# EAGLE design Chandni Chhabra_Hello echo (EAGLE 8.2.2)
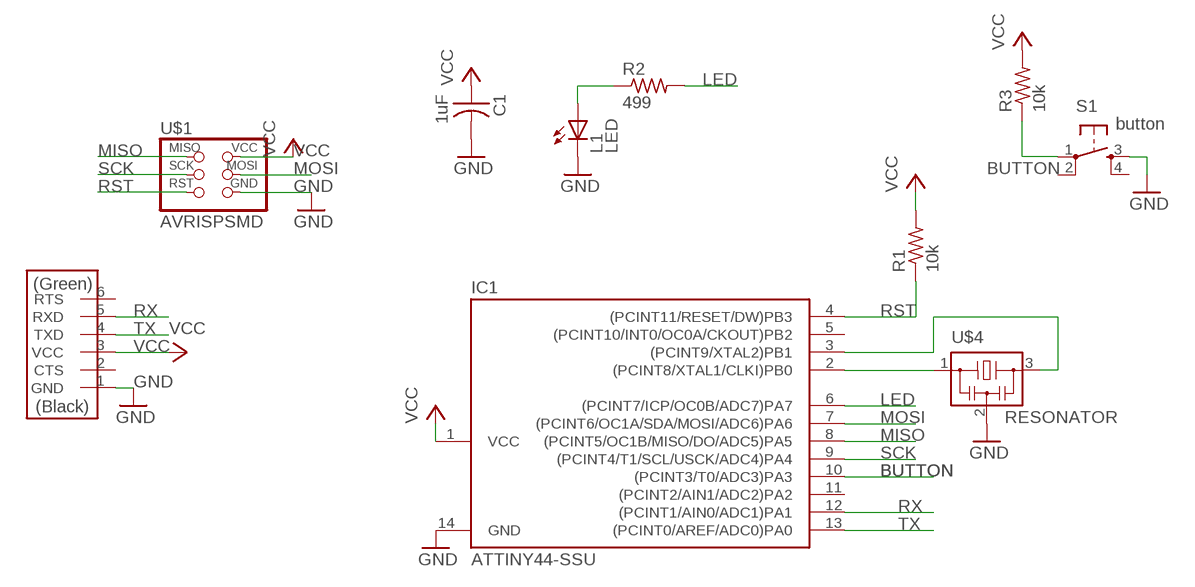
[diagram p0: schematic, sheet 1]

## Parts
C1  1uF  CAP-US1206FAB  [C1206FAB]
IC1  ATTINY44-SSU  [SOIC14]
L1  LED  [LED1206]
R1  10k  RES-US1206FAB  [R1206FAB]
R2  499  RES-US1206FAB  [R1206FAB]
R3  10k  RES-US1206FAB  [R1206FAB]
S1  button  6MM_SWITCH6MM_SWITCH  [6MM_SWITCH]
U$1  AVRISPSMD  [2X03SMD]
U$2  FTDI-SMD-HEADER  [1X06SMD]
U$4  RESONATOR  [EFOBM]

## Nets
BUTTON: IC1.10((PCINT3/T0/ADC3)PA3) R3.1 S1.1(P)
GND: C1.2 IC1.14(GND) L1.2(C) S1.3(S) U$1.6(GND) U$2.1(GND) U$4.2
LED: IC1.6((PCINT7/ICP/OC0B/ADC7)PA7) R2.2
MISO: IC1.8((PCINT5/OC1B/MISO/DO/ADC5)PA5) U$1.1(MISO)
MOSI: IC1.7((PCINT6/OC1A/SDA/MOSI/ADC6)PA6) U$1.4(MOSI)
N$1: IC1.2((PCINT8/XTAL1/CLKI)PB0) U$4.1
N$2: IC1.3((PCINT9/XTAL2)PB1) U$4.3
N$3: L1.1(A) R2.1
RST: IC1.4((PCINT11/RESET/DW)PB3) R1.1 U$1.5(RST)
RX: IC1.12((PCINT1/AIN0/ADC1)PA1) U$2.5(RXD)
SCK: IC1.9((PCINT4/T1/SCL/USCK/ADC4)PA4) U$1.3(SCK)
TX: IC1.13((PCINT0/AREF/ADC0)PA0) U$2.4(TXD)
VCC: C1.1 IC1.1(VCC) R1.2 R3.2 U$1.2(VCC) U$2.3(VCC)
Unconnected: IC1.5((PCINT10/INT0/OC0A/CKOUT)PB2) IC1.11((PCINT2/AIN1/ADC2)PA2) S1.2(P1) S1.4(S1) U$2.2(CTS) U$2.6(RTS)

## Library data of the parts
C1 = fab:CAP-US
IC1 = fab:ATTINY44
L1 = fab:LED: LED
R1-R3 = fab:RES-US: Resistor (US Symbol)
S1 = fab:6MM_SWITCH: OMRON SWITCH
U$1 = fab:AVRISP
U$2 = fab:FTDI-SMD-HEADER
U$4 = fab:RESONATOR

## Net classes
0 default: width 0.032 mm, clearance 0.4 mm

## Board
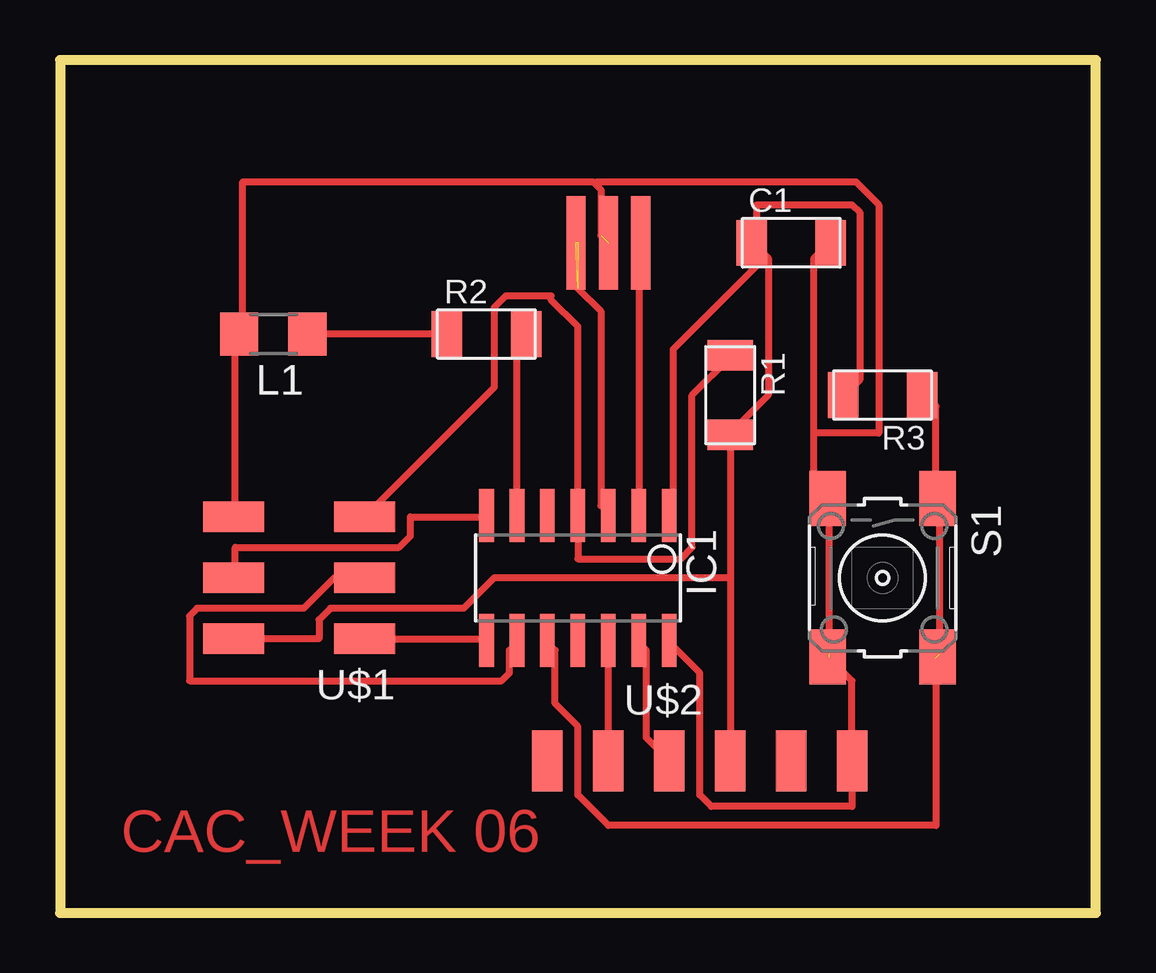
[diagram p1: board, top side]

Size 43.18 x 35.56 mm. Coordinates in mm from the lower left corner, seen from the top.
Outline: 43.18,35.56 0,35.56 0,0 43.18,0 43.18,35.56
Copper layers (1*16): Top 0.035mm / dielectric 1.5mm / Bottom 0.035mm
Design rules "fab *": minimum track width 0.3mm, minimum drill 32mil, track to track 0.4mm, track to pad 0.315mm, pad to pad 0.315mm, via to via 0.315mm, smd to smd 0.315mm, copper to edge 40mil, drill to drill 16mil, minimum pad ring 10mil, minimum via ring 8mil, stop-mask expansion 4mil, vias tented up to drill 0mil, thermal gap 10mil

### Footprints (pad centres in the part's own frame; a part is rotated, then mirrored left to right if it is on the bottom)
C1206FAB = smd 1.27 x 1.905: 1 -1.651,0; 2 1.651,0
SOIC14 = smd 0.61 x 2.21: 1 -3.81,-2.603; 2 -2.54,-2.603; 3 -1.27,-2.603; 4 0,-2.603; 5 1.27,-2.603; 6 2.54,-2.603; 7 3.81,-2.603; 8 3.81,2.603; 9 2.54,2.603; 10 1.27,2.603; 11 0,2.603; 12 -1.27,2.603; 13 -2.54,2.603; 14 -3.81,2.603
LED1206 = smd 1.6 x 1.803: 1 -1.422,0; 2 1.422,0
R1206FAB = smd 1.27 x 1.905: 1 -1.651,0; 2 1.651,0
6MM_SWITCH = smd 2.286 x 1.524: 1 -3.302,2.286; 2 3.302,2.286; 3 -3.302,-2.286; 4 3.302,-2.286
2X03SMD = smd 2.54 x 1.27: 1 -2.54,2.54; 2 2.92,2.54; 3 -2.54,0; 4 2.92,0; 5 -2.54,-2.54; 6 2.92,-2.54
1X06SMD = smd 2.54 x 1.27: 1 0,6.35; 2 0,3.81; 3 0,1.27; 4 0,-1.27; 5 0,-3.81; 6 0,-6.35
EFOBM = smd 0.8 x 3.9: 1 -1.35,0; 2 0,0; 3 1.35,0

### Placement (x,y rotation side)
C1  30.48,27.94 0 top
IC1  21.59,13.97 180 top
L1  8.89,24.13 180 top
R1  27.94,21.59 270 top
R2  17.78,24.13 0 top
R3  34.29,21.59 180 top
S1  34.29,13.97 270 top
U$1  10.16,13.97 180 top
U$2  26.67,6.35 270 top
U$4  22.86,27.94 180 top

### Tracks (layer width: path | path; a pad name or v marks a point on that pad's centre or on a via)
BUTTON  (1 unrouted)
  Top 0.3: R3.1 36.04,21.59 36.51,21.11 36.51,17.3 S1.1 36.67,17.14 36.67,10.79 | 36.51,10.64 36.51,3.65 22.86,3.65 21.59,4.92 21.59,7.78 20.64,8.73 20.64,10.95 20.32,11.27 IC1.10
GND  (2 unrouted)
  Top 0.3: 31.43,20 31.43,17.78 31.91,17.3 S1.3 32.07,17.14 32.07,10.79 | 31.43,20 31.43,27.3 32.07,27.94 C1.2 | IC1.14 25.4,11.27 26.67,10 26.67,4.92 27.15,4.45 33.02,4.45 U$2.1 33.02,9.68 32.07,10.64 | U$1.6 7.3,16.51 7.3,24.13 L1.2 7.62,24.13 7.62,30.48 22.23,30.48 22.3,30.4 | 22.54,28.26 22.54,30.16 22.3,30.4 | 31.43,20 34.13,20 34.13,29.53 33.18,30.48 22.38,30.48 22.3,30.4
LED
  Top 0.3: IC1.6 19.05,23.81 19.37,24.13 R2.2
MISO
  Top 0.3: U$1.1 17.78,11.43 IC1.8
MOSI
  Top 0.3: IC1.7 17.78,16.51 14.61,16.51 14.61,15.72 14.13,15.24 7.3,15.24 7.3,13.97 U$1.4
N$1
  Top 0.3: IC1.2 24.13,27.94 U$4.1
N$2  (3 unrouted)
  Top 0.3: 21.59,26.03 22.54,25.08 22.54,16.99 22.86,16.67 IC1.3
N$3
  Top 0.3: R2.1 L1.1
RST
  Top 0.3: R1.1 27.94,23.18 26.35,21.59 26.35,15.24 25.88,14.76 21.59,14.76 IC1.4 21.59,24.45 20.48,25.56 20.48,25.72 18.57,25.72 18.1,25.24 18.1,21.91 U$1.5
RX
  Top 0.3: U$2.5 IC1.12
SCK
  Top 0.3: U$1.3 11.43,13.97 10.16,12.7 5.72,12.7 5.4,12.38 5.4,9.68 18.42,9.68 18.73,10 18.73,10.95 19.05,11.27 IC1.9
TX
  Top 0.3: U$2.4 24.45,7.3 24.45,10.95 24.13,11.27 IC1.13
VCC
  Top 0.3: C1.1 28.89,27.94 29.53,27.3 29.53,21.59 27.94,20 R1.2 27.94,13.97 | R3.2 32.7,21.59 33.34,22.22 33.34,29.21 33.02,29.53 29.05,29.53 29.05,27.94 C1.1 | IC1.1 25.4,16.67 25.56,16.83 25.56,23.49 29.37,27.3 C1.1 | U$1.2 10.8,11.43 10.8,12.22 11.27,12.7 16.83,12.7 18.1,13.97 27.94,13.97 | 27.94,13.97 U$2.3

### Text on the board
Top: CAC_WEEK 06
